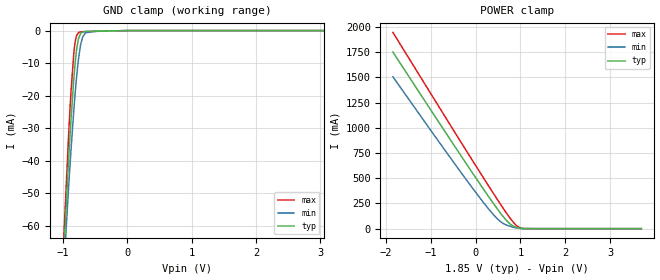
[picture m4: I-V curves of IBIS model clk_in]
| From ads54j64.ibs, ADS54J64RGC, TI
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|   clk_in Model
[Model]   clk_in
Model_type   Input
Vinl = 0.555
Vinh = 1.295
|   typ   min   max
|   (nom PVT)   (fast PVT)   (slow PVT)
C_comp   8.695e-13   6.095e-13   1.035e-12
| Where nom  PVT is Nominal Process, 1.85V, 27C
|   Fast PVT is Strong Process,  1.9V, -40C
|   Slow PVT is Weak Process,   1.8V, 125C
[Voltage Range]   1.85   1.8   1.9
|Junction Temperature
[Temperature Range]   27   125   -40
[Power Clamp Reference]   1.85   1.8   1.9
[GND Clamp Reference]   0   0   0
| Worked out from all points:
|   GND clamp passes 1 mA (typ) near -0.73 V on its own axis
[GND Clamp]
|   Voltage   I(typ)   I(min)   I(max)
-1.85V    -469.1mA   -437.1mA   -490.5mA
-1.001V   -72.29mA   -76.79mA   -68.14mA
-912.1mV  -38.77mA   -47.28mA   -30.94mA
-878.8mV  -27.69mA   -37.1mA    -19.09mA
-834.4mV  -14.89mA   -24.63mA   -7mA
-806.6mV  -8.614mA   -17.74mA   -2.766mA
-762.2mV  -2.556mA   -8.854mA   -646.3uA
-723.4mV  -787.3uA   -3.895mA   -383.4uA
-695.6mV  -428.7uA   -1.963mA   -340.5uA
-651.2mV  -275.8uA   -665.7uA   -310.3uA
-457mV    -176.1uA   -149.6uA   -216.6uA
3.7V      0A         0A         0A
[POWER Clamp]
|   Voltage   I(typ)   I(min)   I(max)
-1.85V    1.752A     1.507A     1.948A
-451.4mV  805.6mA    632.9mA    945.5mA
-1.85mV   506.6mA    361.2mA    627mA
303.4mV   308.4mA    187.4mA    413.5mA
475.4mV   200.9mA    101.9mA    295.3mA
603.1mV   126mA      55mA       209.6mA
786.3mV   40.58mA    21.02mA    93.86mA
925mV     11.12mA    6.17mA     25.95mA
1.003V    3.096mA    1.702mA    7.208mA
1.097V    418.8uA    347uA      631.7uA
3.7V      0A         0A         0A
